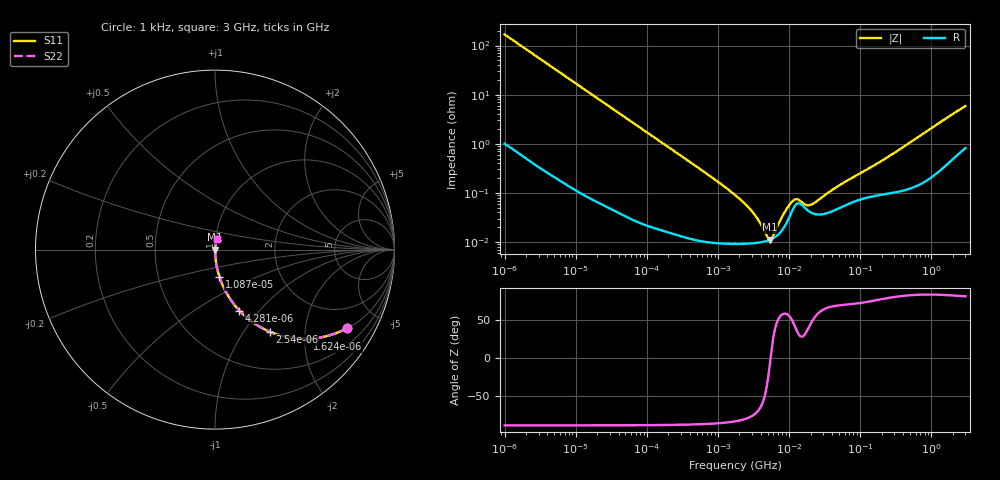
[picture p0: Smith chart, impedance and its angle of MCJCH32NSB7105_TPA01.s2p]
! MCJCH32NSB7105_TPA01  S-PARAMETER MODEL  ( Standard Model )
! Model Generated by TAIYO YUDEN Corporation (http://www.ty-top.com)
! Version 1.0
! TAIYO YUDEN Control No. 220601
! Copyright(c) 2015 TAIYO YUDEN CO.,LTD. All Rights Reserved.
! Product Description (link to TY-COMPAS)
! https://ds.yuden.co.jp/TYCOMPAS/or/detail?pn=MCJCH32NSB7105KTPA01&u=M
! Products Name : Multilayer Ceramic Capacitors
! Characteristics :
!  Capacitance : 1 [uF] , Rated Voltage : 100 [V] , TCC : X7R
!  Case Size : 3.2 x 2.5 / 0.126 x 0.098 [mm/inch] , Thickness : 1.9 / 0.075 [mm/inch]
!  (Conditions: Temperature = 25 [degC] , DC Bias Voltage = 0 [V])
! External Node Assignments :
!  1  o---| |---o  2
! GND o---------o GND
! Frequency Range : 1kHz  -  3GHz  [ 401 STEP ]
# MHZ S RI R 50
! Freq[MHz].  S11 Real  S11 Imag  S21 Real  S21 Imag  S12 Real  S12 Imag  S22 Real  S22 Imag
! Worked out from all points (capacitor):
!   401 points, 1 kHz to 3 GHz, reference 50 ohm
!   read as one part in series: C = 947 nF near 1.077 kHz
!   lowest |Z| = 11.3 mohm at 5.301 MHz (marker M1)
!   series resonance near 5.47 MHz, so ESL is about 890 pH
!   S11 on the Smith chart (normalised r, x): 1 kHz: 1.02, -3.36; 1.624 kHz: 1.01, -2.07; 2.54 kHz: 1.01, -1.33; 4.281 kHz: 1.00, -0.79; 10.87 kHz: 1.00, -0.31; 3 GHz: 1.02, +0.12
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0.001  0.7368 -0.4374  0.2632 0.4374  0.2632 0.4374  0.7368 -0.4374
0.001624  0.5175 -0.4967  0.4825 0.4967  0.4825 0.4967  0.5175 -0.4967
0.00254  0.3066 -0.4581  0.6934 0.4581  0.6934 0.4581  0.3066 -0.4581
0.004281  0.1361 -0.3398  0.8639 0.3398  0.8639 0.3398  0.1361 -0.3398
0.010873  0.0247 -0.1518  0.9753 0.1518  0.9753 0.1518  0.0247 -0.1518
0.01216  0.0199 -0.1364  0.9801 0.1364  0.9801 0.1364  0.0199 -0.1364
0.033275  0.00305 -0.051  0.9969 0.051  0.9969 0.051  0.00305 -0.051
0.147855  0.000313 -0.0116  0.9997 0.0116  0.9997 0.0116  0.000313 -0.0116
1.732051  9.24e-05 -0.000905  0.9999 0.000905  0.9999 0.000905  9.24e-05 -0.000905
3.14518  9.47e-05 -0.000376  0.9999 0.000376  0.9999 0.000376  9.47e-05 -0.000376
3.789741  9.78e-05 -0.000245  0.9999 0.000245  0.9999 0.000245  9.78e-05 -0.000245
4.919932  0.000106 -7.09e-05  0.9999 7.09e-05  0.9999 7.09e-05  0.000106 -7.09e-05
5.30084  0.000111 -2.12e-05  0.9999 2.12e-05  0.9999 2.12e-05  0.000111 -2.12e-05
5.928204  0.000119 5.51e-05  0.9999 -5.51e-05  0.9999 -5.51e-05  0.000119 5.51e-05
8.291982  0.00019 0.000312  0.9998 -0.000312  0.9998 -0.000312  0.00019 0.000312
11.1738  0.00045 0.000513  0.9996 -0.000513  0.9996 -0.000513  0.00045 0.000513
12.97096  0.000608 0.000426  0.9994 -0.000426  0.9994 -0.000426  0.000608 0.000426
17.47891  0.000465 0.000323  0.9995 -0.000323  0.9995 -0.000323  0.000465 0.000323
21.06097  0.000387 0.000446  0.9996 -0.000446  0.9996 -0.000446  0.000387 0.000446
49.64928  0.000485 0.00132  0.9995 -0.00132  0.9995 -0.00132  0.000485 0.00132
256.0921  0.001 0.00554  0.999 -0.00554  0.999 -0.00554  0.001 0.00554
3000  0.0114 0.057  0.9886 -0.057  0.9886 -0.057  0.0114 0.057
